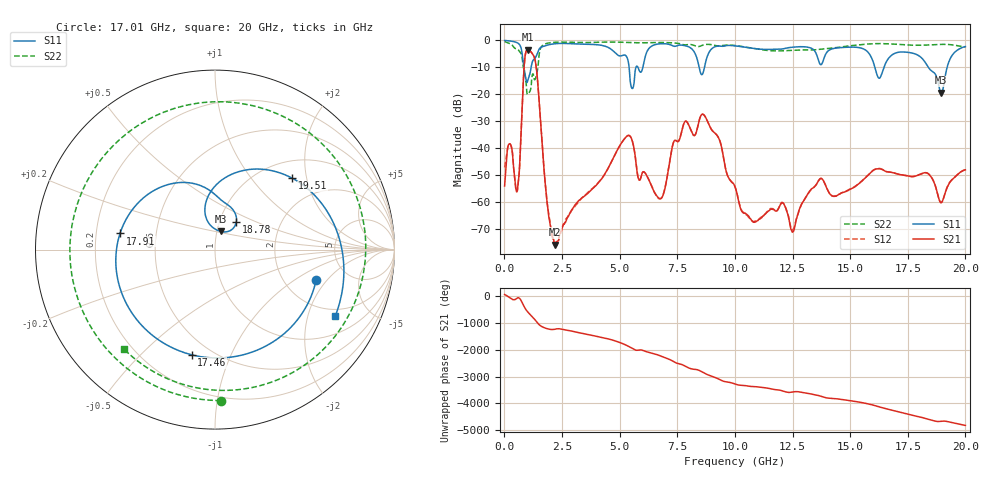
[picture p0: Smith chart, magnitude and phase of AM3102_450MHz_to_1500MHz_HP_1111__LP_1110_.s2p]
!Agilent Technologies,E8364B,MY43040894,A.07.50.67
!Agilent E8364B: A.07.50.67
!Date: Thursday, January 11, 2018 06:52:25
!Correction: S11(Full 2 Port(1,2))
!S21(Full 2 Port(1,2))
!S12(Full 2 Port(1,2))
!S22(Full 2 Port(1,2))
!S2P File: Measurements: S11, S21, S12, S22:
# Hz S  dB  R 50
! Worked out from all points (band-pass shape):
!   1601 points, 10 MHz to 20 GHz, reference 50 ohm
!   highest |S21| = -3.51 dB at 1.022 GHz (marker M1); lowest = -75.8 dB at 2.184 GHz (marker M2)
!   |S21| within 3 dB of the highest: 889.7 MHz to 1.306 GHz (416.8 MHz wide, 38 % of centre)
!   lowest |S11| = -19.5 dB at 18.95 GHz (marker M3), VSWR 1.24, Z = 52.1 + j10.7 ohm
!   |S11| at or under -10 dB: 844.2 MHz to 1.162 GHz (317.5 MHz wide, 31.7 % of centre); 16.07 GHz to 16.47 GHz (396.2 MHz wide, 2.43 % of centre); 18.39 GHz to 19.21 GHz (818 MHz wide, 4.35 % of centre)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
!   |S22| runs from -20.1 to -0.5 dB; largest |S21 - S12| = 0.0025
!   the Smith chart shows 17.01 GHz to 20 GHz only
!   S11 on the Smith chart (normalised r, x): 17.01 GHz: 3.00, -1.53; 17.46 GHz: 0.39, -0.72; 17.91 GHz: 0.30, +0.08; 18.78 GHz: 1.20, +0.39; 19.51 GHz: 1.36, +1.65; 20 GHz: 1.69, -3.02
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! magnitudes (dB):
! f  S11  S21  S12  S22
! 10 MHz  -0.1  -54.0  -47.1  -0.5
! 234.9 MHz  -0.3  -38.4  -38.4  -1.2
! 572.2 MHz  -1.0  -55.0  -55.3  -3.3
! 1.022 GHz  -14.7  -3.5  -3.5  -19.8
! 1.372 GHz  -6.0  -9.3  -9.3  -13.6
! 1.847 GHz  -1.8  -59.6  -59.6  -1.1
! 2.184 GHz  -1.3  -75.8  -76.2  -0.7
! 3.346 GHz  -1.4  -58.6  -58.6  -0.8
! 5.382 GHz  -8.3  -35.3  -35.3  -0.8
! 6.682 GHz  -1.4  -58.4  -58.6  -0.8
! 8.606 GHz  -12.4  -27.4  -27.4  -1.8
! 10.01 GHz  -2.1  -54.3  -54.3  -1.9
! 12.5 GHz  -2.6  -71.1  -70.3  -3.7
! 13.34 GHz  -3.1  -55.0  -55.2  -3.6
! 16.68 GHz  -6.6  -48.8  -48.8  -1.3
! 17.01 GHz  -4.6  -49.5  -49.5  -1.5
! 17.46 GHz  -4.4  -50.2  -50.2  -1.8
! 17.91 GHz  -5.4  -50.1  -50.2  -1.9
! 18.78 GHz  -14.2  -56.4  -56.5  -1.6
! 18.95 GHz  -19.5  -60.2  -60.2  -1.5
! 19.51 GHz  -4.6  -51.0  -51.0  -1.8
! 20 GHz  -2.3  -48.0  -48.0  -2.5
